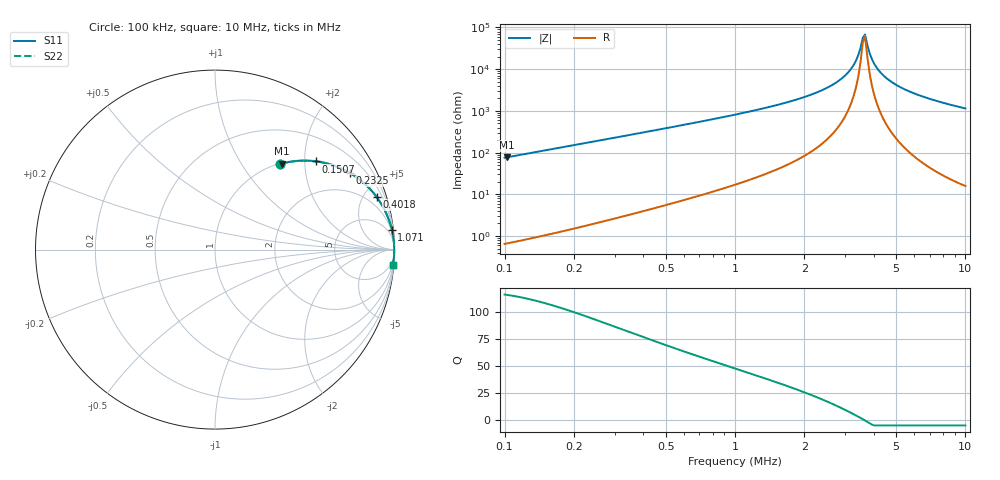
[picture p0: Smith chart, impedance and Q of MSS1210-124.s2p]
# MHz S MA R 50
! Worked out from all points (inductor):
!   203 points, 100 kHz to 10 MHz, reference 50 ohm
!   read as one part in series: L = 120 uH near 102.3 kHz
!   highest Q = 116 at 102.3 kHz (marker M1), where L = 120 uH
!   self-resonance near 3.585 MHz
!   S11 on the Smith chart (normalised r, x): 100 kHz: 1.01, +1.51; 150.7 kHz: 1.02, +2.28; 232.5 kHz: 1.04, +3.52; 401.8 kHz: 1.08, +6.12; 1.071 MHz: 1, +18; 10 MHz: 1, -23
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0.1  0.5999 52.7  0.795 -36.9  0.795 -36.9  0.5999 52.7
0.102306  0.6085 52.0  0.7883 -37.5  0.7883 -37.5  0.6085 52.0
0.1507363  0.7477 41.1  0.6571 -48.4  0.6571 -48.4  0.7477 41.1
0.2324538  0.8653 29.5  0.4922 -59.9  0.4922 -59.9  0.8653 29.5
0.4017542  0.9469 18.0  0.3093 -71.2  0.3093 -71.2  0.9469 18.0
0.6787083  0.9796 10.7  0.1852 -78.4  0.1852 -78.4  0.9796 10.7
1.070787  0.9912 6.5  0.1125 -82.3  0.1125 -82.3  0.9912 6.5
1.768173  0.9964 3.3  0.05733 -84.8  0.05733 -84.8  0.9964 3.3
2.489084  0.998 1.6  0.02846 -85.1  0.02846 -85.1  0.998 1.6
2.919756  0.9984 0.9  0.01631 -83.8  0.01631 -83.8  0.9984 0.9
3.19853  0.9985 0.5  0.009586 -80.8  0.009586 -80.8  0.9985 0.5
3.424944  0.9986 0.3  0.004674 -72.3  0.004674 -72.3  0.9986 0.3
3.584722  0.9986 0.1  0.001778 -39.2  0.001778 -39.2  0.9986 0.1
3.667384  0.9986 -0.0  0.001468 21.6  0.001468 21.6  0.9986 -0.0
3.838472  0.9987 -0.2  0.004098 70.7  0.004098 70.7  0.9987 -0.2
3.926986  0.9987 -0.3  0.005699 76.2  0.005699 76.2  0.9987 -0.3
4.110185  0.9987 -0.5  0.008985 81.1  0.008985 81.1  0.9987 -0.5
4.502621  0.9986 -0.9  0.0157 84.5  0.0157 84.5  0.9986 -0.9
5.162633  0.9984 -1.5  0.02607 85.8  0.02607 85.8  0.9984 -1.5
6.787083  0.9977 -2.8  0.04849 85.9  0.04849 85.9  0.9977 -2.8
8.524974  0.9964 -4.0  0.06981 85.1  0.06981 85.1  0.9964 -4.0
10  0.995 -5.0  0.08676 84.2  0.08676 84.2  0.995 -5.0
